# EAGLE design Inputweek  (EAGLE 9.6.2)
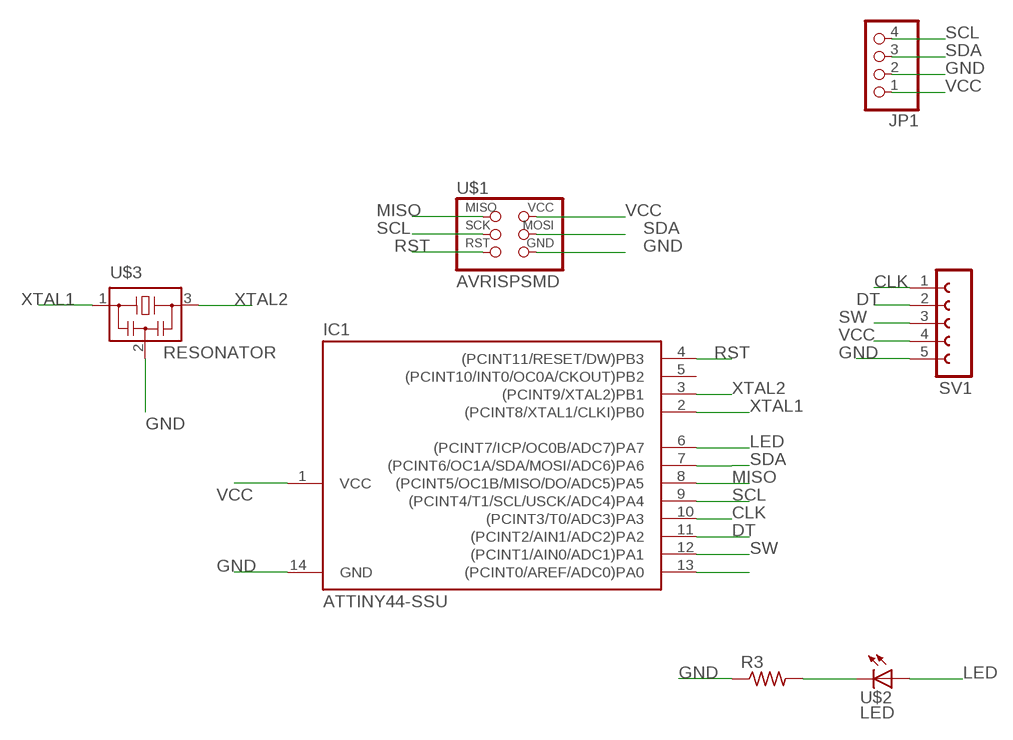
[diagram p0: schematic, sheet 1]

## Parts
IC1  ATTINY44-SSU  [SOIC14]
JP1  PINHD-1X4  [1X04]
R3  RES-US1206  [R1206]
SV1  FE05-1  [FE05-1]
U$1  AVRISPSMD  [2X03SMD]
U$2  LED  [LED1206]
U$3  RESONATOR  [EFOBM]

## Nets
CLK: IC1.10((PCINT3/T0/ADC3)PA3) SV1.1
DT: IC1.11((PCINT2/AIN1/ADC2)PA2) SV1.2
GND: IC1.14(GND) JP1.2 R3.1 SV1.5 U$1.6(GND) U$3.2
LED: IC1.6((PCINT7/ICP/OC0B/ADC7)PA7) U$2.1(A)
MISO: IC1.8((PCINT5/OC1B/MISO/DO/ADC5)PA5) U$1.1(MISO)
N$2: R3.2 U$2.2(C)
N$14: IC1.13((PCINT0/AREF/ADC0)PA0)
RST: IC1.4((PCINT11/RESET/DW)PB3) U$1.5(RST)
SCL: IC1.9((PCINT4/T1/SCL/USCK/ADC4)PA4) JP1.4 U$1.3(SCK)
SDA: IC1.7((PCINT6/OC1A/SDA/MOSI/ADC6)PA6) JP1.3 U$1.4(MOSI)
SW: IC1.12((PCINT1/AIN0/ADC1)PA1) SV1.3
VCC: IC1.1(VCC) JP1.1 SV1.4 U$1.2(VCC)
XTAL1: IC1.2((PCINT8/XTAL1/CLKI)PB0) U$3.1
XTAL2: IC1.3((PCINT9/XTAL2)PB1) U$3.3
Unconnected: IC1.5((PCINT10/INT0/OC0A/CKOUT)PB2)

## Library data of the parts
IC1 = fab:ATTINY44
JP1 = pinhead:PINHD-1X4: PIN HEADER
R3 = fab:RES-US: Resistor (US Symbol)
SV1 = con-lsta:FE05-1: FEMALE HEADER; OC_FARNELL: unknown; OC_NEWARK: unknown
U$1 = fab:AVRISP
U$2 = fab:LED: LED
U$3 = fab:RESONATOR

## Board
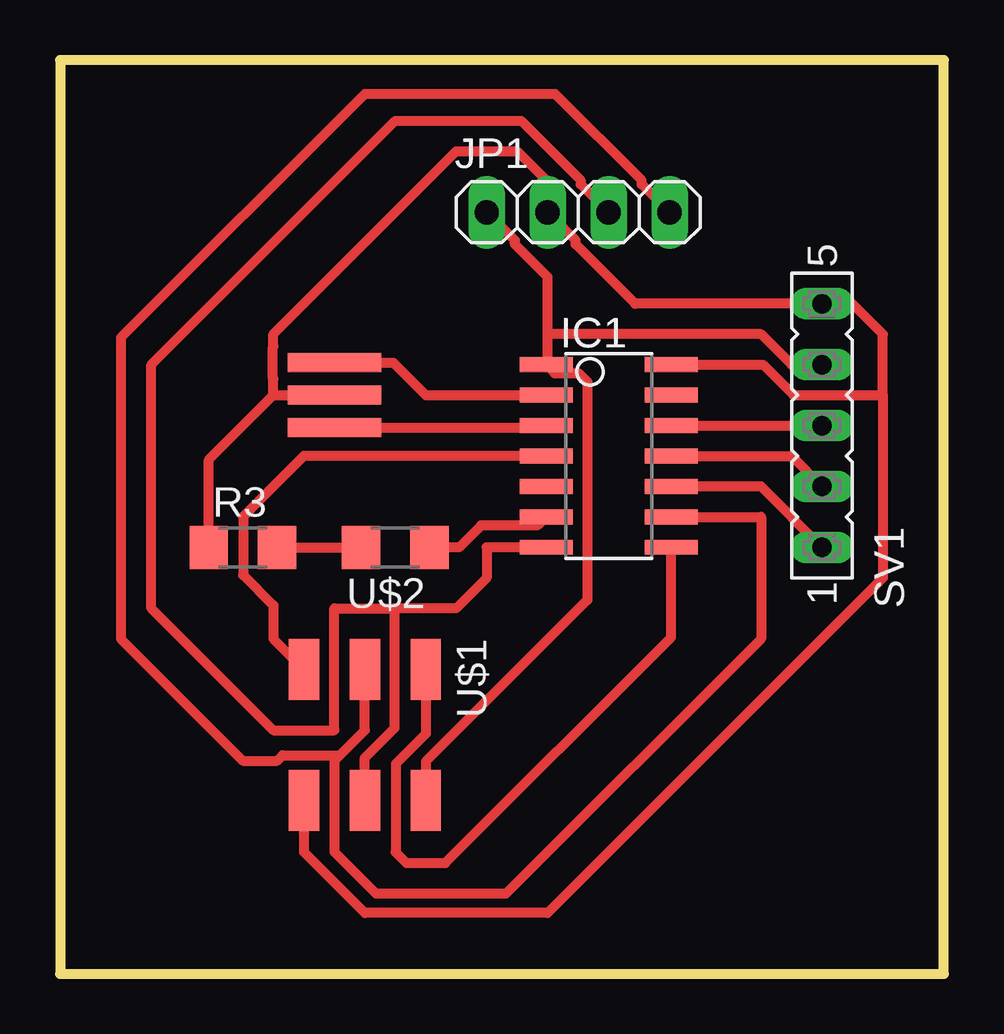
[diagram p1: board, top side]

Size 36.83 x 38.1 mm. Coordinates in mm from the lower left corner, seen from the top.
Outline: 36.83,38.1 0,38.1 0,0 36.83,0 36.83,38.1
Copper layers (1*16): Top 0.035mm / dielectric 1.5mm / Bottom 0.035mm
Design rules "default *": minimum track width 16mil, minimum drill 0.35mm, track to track 16mil, track to pad 16mil, pad to pad 16mil, via to via 16mil, smd to smd 16mil, copper to edge 40mil, drill to drill 16mil, minimum pad ring 10mil, minimum via ring 8mil, stop-mask expansion 4mil, vias tented up to drill 0mil, thermal gap 10mil

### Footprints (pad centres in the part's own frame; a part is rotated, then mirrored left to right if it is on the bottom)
SOIC14 = smd 0.61 x 2.21: 1 -3.81,-2.603; 2 -2.54,-2.603; 3 -1.27,-2.603; 4 0,-2.603; 5 1.27,-2.603; 6 2.54,-2.603; 7 3.81,-2.603; 8 3.81,2.603; 9 2.54,2.603; 10 1.27,2.603; 11 0,2.603; 12 -1.27,2.603; 13 -2.54,2.603; 14 -3.81,2.603
1X04 = drill 1.016 long: 1 -3.81,0; 2 -1.27,0; 3 1.27,0; 4 3.81,0
R1206 = smd 1.6 x 1.803: 1 -1.422,0; 2 1.422,0
FE05-1 = drill 0.813 long: 1 -5.08,0; 2 -2.54,0; 3 0,0; 4 2.54,0; 5 5.08,0
2X03SMD = smd 2.54 x 1.27: 1 -2.54,2.54; 2 2.92,2.54; 3 -2.54,0; 4 2.92,0; 5 -2.54,-2.54; 6 2.92,-2.54
LED1206 = smd 1.6 x 1.803: 1 -1.422,0; 2 1.422,0
EFOBM = smd 0.8 x 3.9: 1 -1.35,0; 2 0,0; 3 1.35,0

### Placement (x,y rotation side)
IC1  22.86,21.59 270 top
JP1  21.59,31.75 0 top
R3  7.62,17.78 0 top
SV1  31.75,22.86 90 top
U$1  12.7,10.16 270 top
U$2  13.97,17.78 180 top
U$3  11.43,24.13 270 top

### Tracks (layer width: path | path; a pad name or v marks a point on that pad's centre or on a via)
CLK
  Top 0.406: SV1.1 29.21,20.32 IC1.10
DT
  Top 0.406: IC1.11 30.48,21.59 SV1.2
GND
  Top 0.406: 20.95,31.12 21.49,30.58 21.49,30.42 23.97,27.94 SV1.5 33.02,27.94 34.29,26.67 34.29,24.13 | 20.95,31.12 JP1.2 | 34.29,24.13 30.56,24.13 29.29,25.4 IC1.14 | 34.29,24.13 34.29,16.51 20.32,2.54 12.7,2.54 10.16,5.08 U$1.6 10.16,7.62 | R3.1 6.2,21.44 8.89,24.13 | 8.89,24.13 U$3.2 | 8.89,24.13 8.89,24.81 8.87,24.83 8.87,26.13 8.89,26.15 8.89,26.67 16.51,34.29 19.05,34.29 20.32,33.02 20.32,30.48 20.95,31.12
LED
  Top 0.406: IC1.6 19.9,18.69 17.54,18.69 16.63,17.78 U$2.1
MISO
  Top 0.406: U$1.1 15.24,10.01 13.99,8.76 13.99,5.11 13.97,5.08 14.43,4.62 16.05,4.62 25.46,14.03 IC1.8
N$2
  Top 0.406: R3.2 U$2.2
RST
  Top 0.406: IC1.4 10.16,21.59 7.63,19.06 7.63,16.63 8.89,15.37 8.89,13.97 U$1.5
SCL
  Top 0.406: JP1.4 24.23,32.92 24.23,33.08 20.63,36.68 12.7,36.68 2.54,26.52 2.54,13.97 7.62,8.89 9.04,8.89 9.27,9.12 11.66,9.12 | U$1.3 12.7,10.16 11.66,9.12 | 11.66,9.12 11.43,8.89 11.43,5.08 13.16,3.35 18.59,3.35 29.21,13.97 29.21,19.05 IC1.9
SDA
  Top 0.406: IC1.7 17.78,17.78 17.78,16.51 16.51,15.24 13.97,15.24 13.95,15.21 | JP1.3 21.69,32.92 21.69,33.08 19.21,35.56 13.97,35.56 3.81,25.4 3.81,15.24 8.89,10.16 11.43,10.16 11.43,15.24 13.92,15.24 13.95,15.21 | U$1.4 12.7,9.01 13.95,10.25 13.95,15.21
SW
  Top 0.406: IC1.12 SV1.3
VCC
  Top 0.406: SV1.4 30.48,25.4 29.21,26.67 20.32,26.67 | JP1.1 18.95,30.58 18.95,30.42 20.32,29.05 20.32,26.67 | 20.32,26.67 20.32,25.46 IC1.1 20.61,25.04 21.61,25.04 21.97,24.69 21.97,15.59 15.24,8.86 U$1.2
XTAL1
  Top 0.406: U$3.1 13.89,25.48 15.24,24.13 IC1.2
XTAL2
  Top 0.406: U$3.3 20.18,22.78 IC1.3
